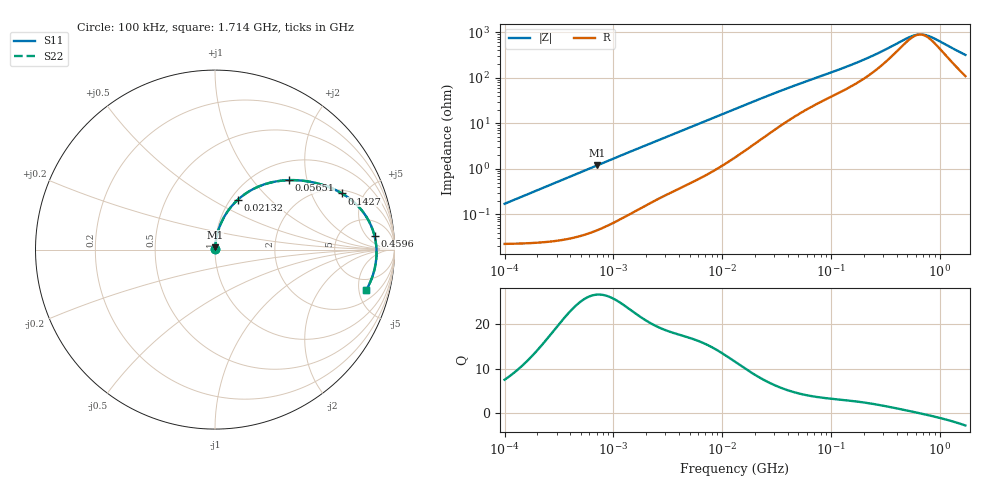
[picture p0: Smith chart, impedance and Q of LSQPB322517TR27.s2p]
! LSQPB322517TR27  S-PARAMETER MODEL  ( General Type )
! Model Generated by TAIYO YUDEN Corporation (http://www.ty-top.com)
! Version 1.0
! TAIYO YUDEN Control No. 100901NG22SB-FKC
! Copyright(c) 2010 TAIYO YUDEN CO.,LTD. All Rights Reserved.
! Product Description (link to TY-COMPAS)
! https://ds.yuden.co.jp/TYCOMPAS/or/detail?pn=LSQPB322517TR27M&u=M
! Products Name : Inductors
! Characteristics :
!  Inductance : 0.27 uH , SRF(min) : 390 MHz , DC Resistance(max) : 0.0286 Ohm
!  Rated Current : Saturation :4500 mA , Temp Rise : 2850 mA (40 degC)
!  Case Size : 3.2 x 2.5 / 0.126 x 0.098 [mm/inch] , Thickness : 1.7 / 0.068 [mm/inch]
!  (Conditions: Temperature = 25 degC , DC Bias Current/Voltage = 0A / 0V)
! External Node Assignments :
!  1  o---GGG---o  2
! GND o---------o GND
! Frequency Range : 0.1MHz  -  1713.942084MHz  [ 402 STEP ]
# MHz S RI R 50
! Freq[MHz].  S11 Real  S11 Imag  S21 Real  S21 Imag  S12 Real  S12 Imag  S22 Real  S22 Imag
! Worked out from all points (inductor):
!   401 points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, 100 kHz to 1.714 GHz, reference 50 ohm
!   read as one part in series: L = 270 nH near 105 kHz
!   highest Q = 26.7 at 702.7 kHz (marker M1), where L = 269 nH
!   self-resonance near 652.4 MHz
!   S11 on the Smith chart (normalised r, x): 100 kHz: 1.00, +0.00; 21.32 MHz: 1.08, +0.66; 56.51 MHz: 1.38, +1.57; 142.7 MHz: 2.19, +3.41; 459.6 MHz: 12, +8; 1.714 GHz: 3.18, -6.00
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0.1  0.000228 0.0017  0.9998 -0.0017  0.9998 -0.0017  0.000228 0.0017
0.511911  0.000417 0.00866  0.9996 -0.00866  0.9996 -0.00866  0.000417 0.00866
0.702747  0.000585 0.0119  0.9994 -0.0119  0.9994 -0.0119  0.000585 0.0119
2.620527  0.00407 0.0428  0.9959 -0.0428  0.9959 -0.0428  0.00407 0.0428
6.301564  0.0161 0.0987  0.9839 -0.0987  0.9839 -0.0987  0.0161 0.0987
13.41476  0.0585 0.195  0.9415 -0.195  0.9415 -0.195  0.0585 0.195
21.31562  0.126 0.2766  0.874 -0.2766  0.874 -0.2766  0.126 0.2766
36.4391  0.2657 0.3603  0.7343 -0.3603  0.7343 -0.3603  0.2657 0.3603
56.50638  0.4136 0.3871  0.5864 -0.3871  0.5864 -0.3871  0.4136 0.3871
67.01815  0.4722 0.3854  0.5278 -0.3854  0.5278 -0.3854  0.4722 0.3854
96.59781  0.5925 0.3628  0.4075 -0.3628  0.4075 -0.3628  0.5925 0.3628
142.6682  0.7072 0.3131  0.2928 -0.3131  0.2928 -0.3131  0.7072 0.3131
221.2366  0.8072 0.2311  0.1928 -0.2311  0.1928 -0.2311  0.8072 0.2311
343.0732  0.8681 0.1366  0.1319 -0.1366  0.1319 -0.1366  0.8681 0.1366
459.6282  0.8895 0.0738  0.1105 -0.0738  0.1105 -0.0738  0.8895 0.0738
532.0061  0.8956 0.0429  0.1044 -0.0429  0.1044 -0.0429  0.8956 0.0429
600.9545  0.8986 0.0173  0.1014 -0.0173  0.1014 -0.0173  0.8986 0.0173
662.4933  0.8998 -0.00327  0.1002 0.00327  0.1002 0.00327  0.8998 -0.00327
730.3339  0.8998 -0.024  0.1002 0.024  0.1002 0.024  0.8998 -0.024
866.1965  0.8973 -0.0608  0.1027 0.0608  0.1027 0.0608  0.8973 -0.0608
1410.315  0.8679 -0.1744  0.1321 0.1744  0.1321 0.1744  0.8679 -0.1744
1713.942  0.8436 -0.2243  0.1564 0.2243  0.1564 0.2243  0.8436 -0.2243
